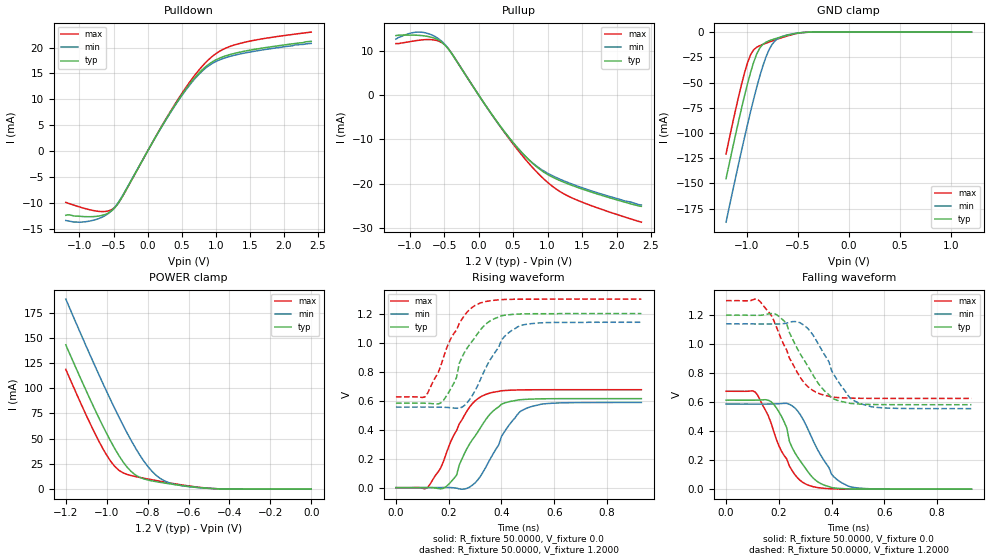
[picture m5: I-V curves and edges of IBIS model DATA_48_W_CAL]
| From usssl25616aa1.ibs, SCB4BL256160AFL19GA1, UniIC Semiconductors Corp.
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|   Model DATA_48_W_CAL
[Model]  DATA_48_W_CAL
Model_type I/O
Polarity   Non-Inverting
Enable   Active-High
Vinl =   0.3800V
Vinh =   0.8200V
Vmeas =  0.6000V
Cref =   5.0000pF
Rref =   50.0000
Vref =   0.6000V
C_comp   1.7430pF   1.7110pF   1.7640pF
[Temperature Range]   25.0000   0.1250k   -40.0000
[Voltage Range]   1.2000V   1.1400V   1.3000V
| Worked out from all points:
|   slope of the pulldown table from 0 to 0.18 V, typ, clamps not added: 43.4 ohm
|   slope of the pullup table from 0 to 0.18 V, typ, clamps not added: 43.8 ohm
|   GND clamp passes 1 mA (typ) near -0.50 V on its own axis
|   POWER clamp passes 1 mA (typ) near -0.51 V on its own axis
|   rising waveform, R_fixture 50.0000, V_fixture 0.0: 20-80 % time 114ps typ, 113ps min, 104ps max; typ from 0 V to 0.614 V
|   rising waveform, R_fixture 50.0000, V_fixture 1.2000: 20-80 % time 100ps typ, 101ps min, 102ps max; typ from 0.582 V to 1.2 V
|   falling waveform, R_fixture 50.0000, V_fixture 0.0: 20-80 % time 96.3ps typ, 102ps min, 97.6ps max; typ from 0.614 V to 0 V
|   falling waveform, R_fixture 50.0000, V_fixture 1.2000: 20-80 % time 118ps typ, 110ps min, 105ps max; typ from 1.2 V to 0.582 V
[Pulldown]
|Voltage   I(typ)   I(min)   I(max)
-1.2V     -12.4mA    -13.4mA    -9.9mA
-1V       -12.59mA   -13.73mA   -10.78mA
-760mV    -12.61mA   -13.23mA   -11.56mA
-600mV    -12.12mA   -12.26mA   -11.63mA
-480mV    -10.93mA   -10.83mA   -10.84mA
-360mV    -8.541mA   -8.428mA   -8.575mA
400mV     8.867mA    8.739mA    9.039mA
680mV     13.98mA    13.78mA    14.44mA
880mV     16.6mA     16.33mA    17.48mA
1.08V     18.08mA    17.74mA    19.46mA
1.32V     19.01mA    18.65mA    20.67mA
2.4V      21.2mA     20.8mA     22.98mA
[Pullup]
|Voltage   I(typ)   I(min)   I(max)
-1.2V     13.4mA     12.6mA     11.6mA
-1V       13.52mA    13.91mA    12.03mA
-840mV    13.42mA    14.18mA    12.4mA
-680mV    13.01mA    13.55mA    12.48mA
-520mV    11.74mA    11.9mA     11.68mA
-400mV    9.531mA    9.603mA    9.587mA
320mV     -7.122mA   -7.211mA   -7.27mA
560mV     -11.8mA    -11.87mA   -12.25mA
800mV     -15.63mA   -15.54mA   -16.65mA
1.08V     -18.58mA   -18.27mA   -20.7mA
1.32V     -20.18mA   -19.88mA   -22.95mA
2.36V     -25.1mA    -24.8mA    -28.67mA
[GND_clamp]
|Voltage   I(typ)   I(min)   I(max)
-1.2V     -145.3mA   -188.5mA   -120.8mA
-1.05V    -76.2mA    -118.2mA   -52.43mA
-990mV    -51.2mA    -91.62mA   -30.39mA
-960mV    -39.9mA    -78.82mA   -22.48mA
-900mV    -21.67mA   -54.7mA    -15mA
-870mV    -15.78mA   -43.66mA   -13.45mA
-810mV    -10.04mA   -24.79mA   -11.07mA
-780mV    -8.658mA   -17.59mA   -9.958mA
-720mV    -6.57mA    -8.545mA   -7.793mA
-630mV    -3.906mA   -3.64mA    -4.741mA
-420mV    -215.4uA   -240.5uA   -235uA
1.2V      1.597nA    22.84nA    1.463nA
[POWER_clamp]
|Voltage   I(typ)   I(min)   I(max)
-1.2V     143mA      188.4mA    118.7mA
-1.1V     97.38mA    141.5mA    73.24mA
-1.04V    71.38mA    114.3mA    48.22mA
-1V       55.04mA    96.69mA    33.64mA
-960mV    40mA       79.65mA    22.42mA
-900mV    21.75mA    55.6mA     14.58mA
-860mV    14.17mA    41.05mA    12.52mA
-800mV    9.133mA    22.79mA    10.12mA
-740mV    6.786mA    10.88mA    7.886mA
-660mV    4.332mA    4.436mA    5.101mA
-520mV    1.103mA    1.063mA    1.274mA
0V        1.597nA    6.003nA    2.16nA
[Ramp]
| variable   typ   min   max
dV/dt_r  0.3682/0.1099n   0.3523/0.1141n   0.4051/0.1060n
dV/dt_f  0.3705/0.1101n   0.3508/0.1127n   0.4045/0.1066n
R_load = 50.0000
[Rising Waveform]
R_fixture= 50.0000
V_fixture= 0.0
V_fixture_min= 0.0
V_fixture_max= 0.0
|time   V(typ)   V(min)   V(max)
0s        0V         0V         0V
120ps     1.127mV    177uV      896.5uV
170ps     -8.205mV   948.1uV    136.8mV
190ps     7.022mV    1.361mV    232.2mV
230ps     87.34mV    -3.222mV   394.5mV
270ps     272.4mV    -4.208mV   531.1mV
340ps     468.3mV    139.4mV    642.4mV
420ps     588.3mV    409.1mV    670.5mV
490ps     608.5mV    543.3mV    674.4mV
930ps     613.7mV    587.1mV    675.2mV
[Rising Waveform]
R_fixture= 50.0000
V_fixture= 1.2000
V_fixture_min= 1.1400
V_fixture_max= 1.3000
|time   V(typ)   V(min)   V(max)
0s        582.5mV    555.3mV    625.9mV
110ps     582.1mV    555.6mV    625.6mV
170ps     583.7mV    554.6mV    838.9mV
220ps     721.7mV    548.8mV    1.064V
250ps     898.1mV    554.4mV    1.161V
280ps     987.7mV    609.7mV    1.229V
320ps     1.087V     744.5mV    1.273V
400ps     1.185V     1.018V     1.296V
470ps     1.197V     1.116V     1.299V
930ps     1.2V       1.14V      1.3V
[Falling Waveform]
R_fixture= 50.0000
V_fixture= 0.0
V_fixture_min= 0.0
V_fixture_max= 0.0
|time   V(typ)   V(min)   V(max)
0s        613.7mV    587.1mV    675.2mV
110ps     613.6mV    586.8mV    670.8mV
170ps     603.9mV    587.3mV    459.5mV
220ps     465mV      591.8mV    232.2mV
250ps     288.7mV    575.7mV    129.5mV
310ps     120.9mV    414.6mV    28.64mV
350ps     47.7mV     262mV      10.21mV
400ps     10.85mV    102.2mV    2.161mV
470ps     1.473mV    16.78mV    271.3uV
930ps     0V         0V         0V
[Falling Waveform]
R_fixture= 50.0000
V_fixture= 1.2000
V_fixture_min= 1.1400
V_fixture_max= 1.3000
|time   V(typ)   V(min)   V(max)
0s        1.2V       1.14V      1.3V
120ps     1.199V     1.139V     1.308V
170ps     1.211V     1.139V     1.203V
200ps     1.192V     1.139V     1.076V
230ps     1.14V      1.145V     958.5mV
280ps     936.5mV    1.148V     774mV
350ps     728.4mV    1V         661.1mV
430ps     608.1mV    728.5mV    631.1mV
500ps     587.6mV    597mV      626.8mV
930ps     582.5mV    555.3mV    625.9mV
